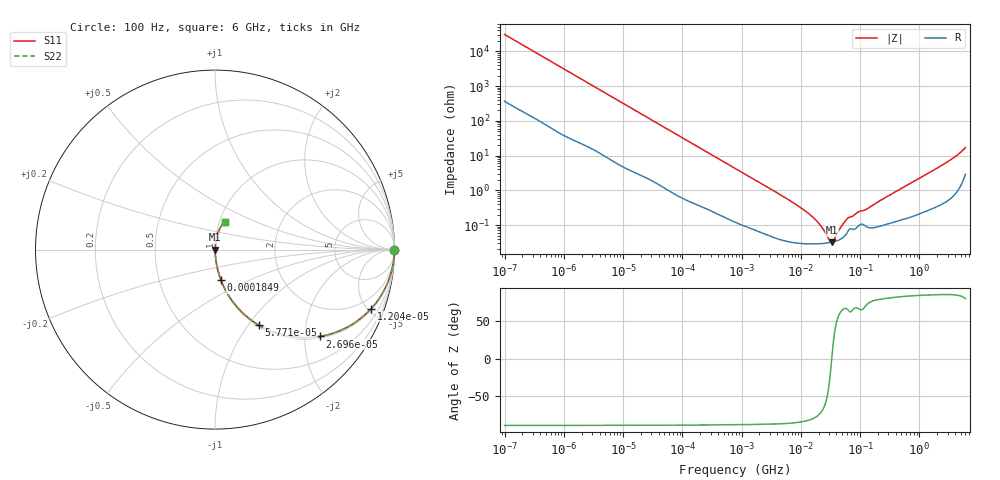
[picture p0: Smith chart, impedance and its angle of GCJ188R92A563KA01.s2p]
!Murata Part Number: GCJ188R92A563KA01
!These Parameters are Measured in Series Mode Connection
!Data Generated on Mar 13, 2026
!  o--ll--o
!Port1  Port2
!  o------o
!Operation Temp=25[degC], DC Bias Voltage=0[V]
!Freq. Start=100[Hz] Stop=6[GHz] 401[Steps]
# Hz S RI R 50
!Freq.(Hz) S11(Real) S11(Imag) S21(Real) S21(Imag) S12(Real) S12(Imag) S22(Real) S22(Imag)
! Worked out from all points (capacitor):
!   401 points, 100 Hz to 6 GHz, reference 50 ohm
!   read as one part in series: C = 52 nF near 109 Hz
!   lowest |Z| = 32.2 mohm at 33.3 MHz (marker M1)
!   series resonance near 33.26 MHz, so ESL is about 440 pH
!   S11 on the Smith chart (normalised r, x): 100 Hz: open; 12.04 kHz: 1.08, -5.27; 26.96 kHz: 1.04, -2.38; 57.71 kHz: 1.02, -1.12; 184.9 kHz: 1.01, -0.35; 6 GHz: 1.06, +0.33
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100  1 -0.00328  5e-05 0.00328  5e-05 0.00328  1 -0.00328
2008  0.995 -0.0639  0.005 0.0639  0.005 0.0639  0.995 -0.0639
5143  0.9719 -0.1581  0.0281 0.1581  0.0281 0.1581  0.9719 -0.1581
12041  0.8705 -0.3282  0.1295 0.3282  0.1295 0.3282  0.8705 -0.3282
26957  0.5838 -0.4841  0.4162 0.4841  0.4162 0.4841  0.5838 -0.4841
40335  0.391 -0.479  0.609 0.479  0.609 0.479  0.391 -0.479
57709  0.2428 -0.4199  0.7572 0.4199  0.7572 0.4199  0.2428 -0.4199
98762  0.1019 -0.2936  0.8981 0.2936  0.8981 0.2936  0.1019 -0.2936
184852  0.0337 -0.1703  0.9663 0.1703  0.9663 0.1703  0.0337 -0.1703
774597  0.00305 -0.0429  0.9969 0.0429  0.9969 0.0429  0.00305 -0.0429
6353432  0.000356 -0.00522  0.9996 0.00522  0.9996 0.00522  0.000356 -0.00522
1.555665e7  0.00029 -0.00174  0.9997 0.00174  0.9997 0.00174  0.00029 -0.00174
2.225763e7  0.000294 -0.000861  0.9997 0.000861  0.9997 0.000861  0.000294 -0.000861
3.045065e7  0.000313 -0.000185  0.9997 0.000185  0.9997 0.000185  0.000313 -0.000185
3.330331e7  0.000322 2.8e-06  0.9997 -2.8e-06  0.9997 -2.8e-06  0.000322 2.8e-06
3.64232e7  0.000334 0.000192  0.9997 -0.000192  0.9997 -0.000192  0.000334 0.000192
4.983056e7  0.00042 0.000897  0.9996 -0.000897  0.9996 -0.000897  0.00042 0.000897
6.233367e7  0.000662 0.00144  0.9993 -0.00144  0.9993 -0.00144  0.000662 0.00144
1.275994e8  0.000909 0.00269  0.9991 -0.00269  0.9991 -0.00269  0.000909 0.00269
3.124326e8  0.00116 0.0071  0.9988 -0.0071  0.9988 -0.0071  0.00116 0.0071
2.562649e9  0.00726 0.0552  0.9927 -0.0552  0.9927 -0.0552  0.00726 0.0552
6e9  0.0531 0.154  0.9469 -0.154  0.9469 -0.154  0.0531 0.154
